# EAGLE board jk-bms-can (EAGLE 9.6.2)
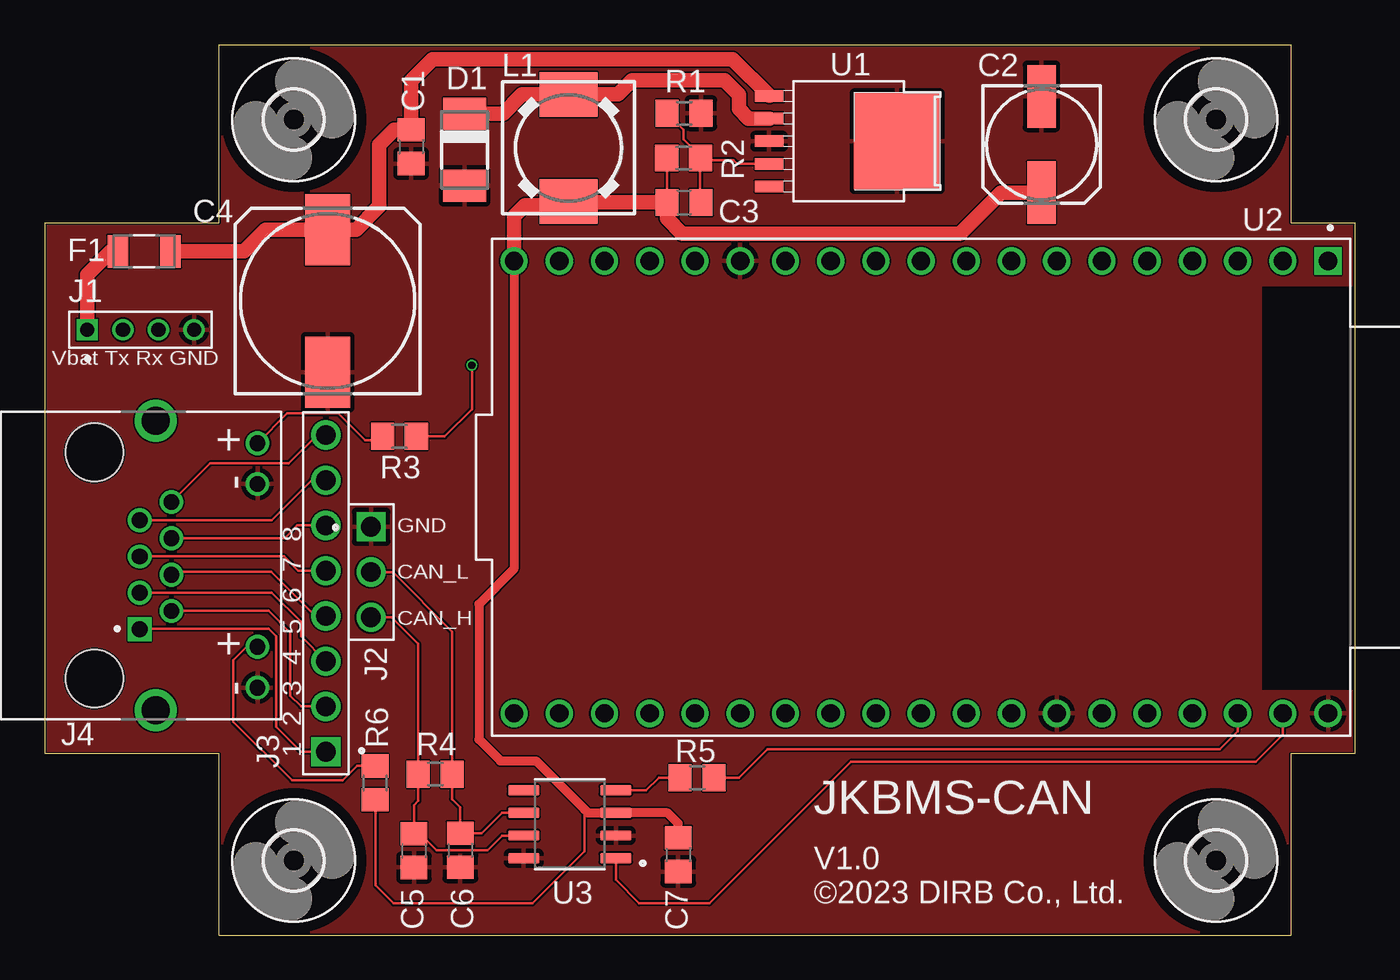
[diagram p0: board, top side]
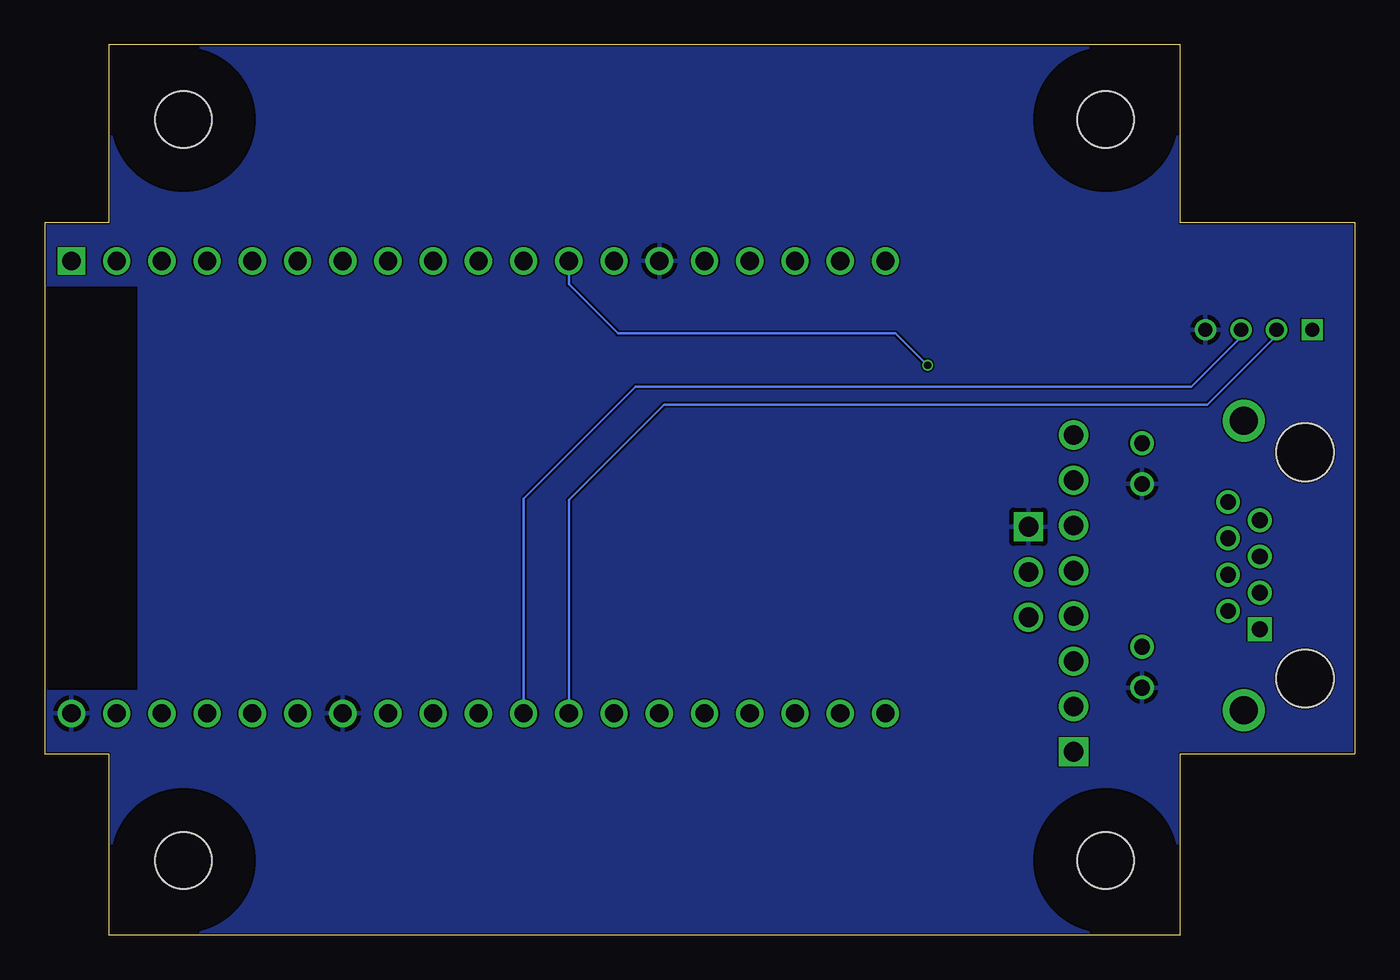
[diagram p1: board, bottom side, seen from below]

Size 73.6 x 50 mm. Coordinates in mm from the lower left corner, seen from the top.
Outline: 9.8,0 70,0 70,10.2 73.6,10.2 73.6,40 70,40 70,50 9.8,50 9.8,40 0,40 0,10.2 9.8,10.2 9.8,0
Copper layers (1*16): Top 0.035mm / dielectric 0.2mm / Bottom 0.035mm
Design rules "jlcpcb-2-layer": minimum track width 3.5mil, minimum drill 0.2mm, track to track 3.5mil, track to pad 5mil, pad to pad 5mil, via to via 5mil, smd to smd 0mil, copper to edge 0.1mm, drill to drill 5mil, minimum pad ring 4mil, minimum via ring 4mil, stop-mask expansion 3mil, vias tented up to drill 100mil, thermal gap 10mil
tRestrict: area 68.4,13.8 to 73.4,36.4
bRestrict: area 68.4,13.8 to 73.4,36.4

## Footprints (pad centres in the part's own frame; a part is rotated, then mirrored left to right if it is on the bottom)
C0805 = smd 1.3 x 1.5: 1 -0.95,0; 2 0.95,0
153CLV-0605 = smd 3.5 x 1.6: + 2.7,0; - -2.7,0
153CLV-1010 = smd 4 x 2.5: + 4,0; - -4,0
DO-214AC = smd 1.8 x 2.4: A 2.025,0; C -2.025,0
FUSC3216X75N = smd 1.16 x 1.82: 1 -1.475,0; 2 1.475,0
3,2 = hole 3.2: 0,0
62000411121 = drill 0.8 square: 1 -3,0 | drill 0.8: 2 -1,0; 3 1,0; 4 3,0
61300311121 = drill 1.1 square: 1 -2.54,0 | drill 1.1: 2 0,0; 3 2.54,0
61300811121 = drill 1.1 square: 1 -8.89,0 | drill 1.1: 2 -6.35,0; 3 -3.81,0; 4 -1.27,0; 5 1.27,0; 6 3.81,0; 7 6.35,0; 8 8.89,0
TE_2-406549-1 = drill 0.89 square: 1 0,0 | drill 0.89: 2 -1.02,1.78; 3 -2.04,0; 4 -3.06,1.78; 5 -4.08,0; 6 -5.1,1.78; 7 -6.12,0; 8 -7.14,1.78; 9 3.28,6.61; 10 0.99,6.61; 11 -8.15,6.61; 12 -10.44,6.61 | drill 1.57: S1 -11.71,0.89; S2 4.55,0.89 | hole 3.25: -9.93,-2.54; 2.77,-2.54
DR74 = smd 2.5 x 3.25: 1 -3,0; 2 3,0
R0805 = smd 1.3 x 1.5: 1 -0.95,0; 2 0.95,0
TO-252-5L = smd 0.65 x 1.6: 1 -2.535,-4.465; 2 -1.265,-4.465; 3 0.005,-4.47; 4 1.275,-4.47; 5 2.545,-4.47 | smd 5.42 x 4.84: 6/GND 0,2.715
MODULE_ESP32-DEVKITC-32U = drill 1.02 square: 1 -12.7,22.85 | drill 1.02: 2 -12.7,20.31; 3 -12.7,17.77; 4 -12.7,15.23; 5 -12.7,12.69; 6 -12.7,10.15; 7 -12.7,7.61; 8 -12.7,5.07; 9 -12.7,2.53; 10 -12.7,-0.01; 11 -12.7,-2.55; 12 -12.7,-5.09; 13 -12.7,-7.63; 14 -12.7,-10.17; 15 -12.7,-12.71; 16 -12.7,-15.25; 17 -12.7,-17.79; 18 -12.7,-20.33; 19 -12.7,-22.87; 20 12.7,-22.87; 21 12.7,-20.33; 22 12.7,-17.79; 23 12.7,-15.25; 24 12.7,-12.71; 25 12.7,-10.17; 26 12.7,-7.63; 27 12.7,-5.09; 28 12.7,-2.55; 29 12.7,-0.01; 30 12.7,2.53; 31 12.7,5.07; 32 12.7,7.61; 33 12.7,10.15; 34 12.7,12.69; 35 12.7,15.23; 36 12.7,17.77; 37 12.7,20.31; 38 12.7,22.85
SOIC127P600X175-8N = smd 1.75 x 0.59: 1 -2.585,1.905; 2 -2.585,0.635; 3 -2.585,-0.635; 4 -2.585,-1.905; 5 2.585,-1.905; 6 2.585,-0.635; 7 2.585,0.635; 8 2.585,1.905

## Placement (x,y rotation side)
C1  100n  [C0805]  20.59,44.28 270 top
C2  100uF/25V  [153CLV-0605]  56,44.4 270 top
C3  33n  [C0805]  35.92,41.15 0 top
C4  33uF/100V  [153CLV-1010]  15.9,35.62 90 top
C5  30p  [C0805]  20.75,4.76 270 top
C6  30p  [C0805]  23.35,4.78 270 top
C7  100n  [C0805]  35.59,4.53 270 top
D1  SS210  [DO-214AC]  23.59,44.1 270 top
F1  1206L035YR  [FUSC3216X75N]  5.6,38.4 0 top
H1  MOUNT-HOLE3.2  [3,2]  14,45.8 0 top
H2  MOUNT-HOLE3.2  [3,2]  65.8,45.8 0 top
H3  MOUNT-HOLE3.2  [3,2]  14,4.2 0 top
H4  MOUNT-HOLE3.2  [3,2]  65.8,4.2 0 top
J1  62000411121  [62000411121]  5.4,34 0 top
J2  61300311121  [61300311121]  18.34,20.4 270 top
J3  61300811121  [61300811121]  15.8,19.2 90 top
J4  2-406549-1  [TE_2-406549-1]  5.35,17.19 270 top
L1  470uH/0.5A  [DR74]  29.43,44.21 270 top
R1  10k  [R0805]  35.92,46.15 180 top
R2  30k  [R0805]  35.9,43.65 180 top
R3  10k  [R0805]  19.93,28.02 180 top
R4  120  [R0805]  21.94,9.05 180 top
R5  4K7  [R0805]  36.65,8.85 0 top
R6  10k  [R0805]  18.57,8.56 90 top
U1  XL7015  [TO-252-5L]  45.17,44.59 270 top
U2  ESP32-DEVKITC-32U  [MODULE_ESP32-DEVKITC-32U]  49.24,25.16 270 top
U3  TJA1050T/CM,118  [SOIC127P600X175-8N]  29.5,6.24 180 top

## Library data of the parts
C1-C7 = rcl; SPICEPREFIX: C
D1 = diode
F1 = 1206L035YR; AVAILABILITY: In Stock; CHECK_PRICES: https://www.snapeda.com/parts/1206L035YR/Littelfuse/view-part/?ref=eda; DESCRIPTION: PTC Resettable Fuse 0.35A(hold) 0.75A(trip) 6VDC 100A 0.6W 0.1s 0.3Ohm SMD Solder Pad 1206 T/R; MF: Littelfuse; MP: 1206L035YR; PACKAGE: None; PRICE: None; PURCHASE-URL: https://pricing.snapeda.com/search?q=1206L035YR&ref=eda; SNAPEDA_LINK: https://www.snapeda.com/parts/1206L035YR/Littelfuse/view-part/?ref=snap
H1-H4 = holes
J1 = Headers; CREATED_BY: PCBLayout.com; MANUFACTURER: Würth Elektronik; MPN: 62000411121
J2 = Headers; CREATED_BY: PCBLayout.com; DIGI_KEY_PART_NUMBER: 732-5316-ND; MANUFACTURER: Wurth Electronics Inc.; MPN: 61300311121
J3 = Headers; CREATED_BY: PCBLayout.com; DIGI_KEY_PART_NUMBER: 732-5321-ND; MANUFACTURER: Wurth Electronics Inc.; MPN: 61300811121
J4 = 2-406549-1; AVAILABILITY: In Stock; CENTERLINE_PITCH: 1.02 mm[.04 in]; CHECK_PRICES: https://www.snapeda.com/parts/2-406549-1/TE+Connectivity+AMP+Connectors/view-part/?ref=eda; COMMENT: 2-406549-1; DESCRIPTION: Jack Modular Connector 8p8c (RJ45, Ethernet) 90° Angle (Right) Shielded, EMI Finger Cat5; EU_ROHS_COMPLIANCE: Compliant; MF: TE Connectivity; MP: 2-406549-1; NUMBER_OF_POSITIONS: 8; PACKAGE: None; PRICE: None; PURCHASE-URL: https://pricing.snapeda.com/search?q=2-406549-1&ref=eda; SNAPEDA_LINK: https://www.snapeda.com/parts/2-406549-1/TE+Connectivity+AMP+Connectors/view-part/?ref=snap
L1 = inductors; SPICEPREFIX: L
R1-R6 = rcl; SPICEPREFIX: R
U1 = XL7015; AVAILABILITY: Not in stock; CHECK_PRICES: https://www.snapeda.com/parts/XL7015/XLSEMI/view-part/?ref=eda; DESCRIPTION: 0.8A 150KHz 80V Buck DC to DC; MF: XLSEMI; MP: XL7015; PACKAGE: Package; PRICE: None; SNAPEDA_LINK: https://www.snapeda.com/parts/XL7015/XLSEMI/view-part/?ref=snap
U2 = ESP32-DEVKITC-32U; AVAILABILITY: In Stock; CHECK_PRICES: https://www.snapeda.com/parts/ESP32-DEVKITC-32U/Espressif+Systems/view-part/?ref=eda; DESCRIPTION: ESP32-WROOM-32UE series Transceiver; 802.11 b/g/n (Wi-Fi, WiFi, WLAN), Bluetooth® Smart Ready 4.x Dual Mode Evaluation Board; MF: Espressif Systems; MP: ESP32-DEVKITC-32U; PACKAGE: CUSTOM-38 ESPRESSIF; PRICE: None; PURCHASE-URL: https://pricing.snapeda.com/search?q=ESP32-DEVKITC-32U&ref=eda; SNAPEDA_LINK: https://www.snapeda.com/parts/ESP32-DEVKITC-32U/Espressif+Systems/view-part/?ref=snap
U3 = TJA1050T_CM_118; AVAILABILITY: In Stock; CHECK_PRICES: https://www.snapeda.com/parts/TJA1050T/CM,118/NXP+USA+Inc./view-part/?ref=eda; DESCRIPTION: 1/1 Transceiver Half CANbus 8-SO; MF: NXP USA; MP: TJA1050T/CM,118; PACKAGE: SO-8 NXP Semiconductors; PRICE: None; PURCHASE-URL: https://pricing.snapeda.com/search?q=TJA1050T/CM,118&ref=eda; SNAPEDA_LINK: https://www.snapeda.com/parts/TJA1050T/CM,118/NXP+USA+Inc./view-part/?ref=snap

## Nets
3V3: U2.1
CAN_RXD: R5.1 U3.4
CAN_TXD: U2.37 U3.1
GND: C1.2 C2.- C4.- C5.2 C6.2 C7.2 D1.A J1.4 J2.1 J4.9 J4.11 R1.1 U1.3 U1.6/GND U2.14 U2.32 U2.38 U3.2 U3.8
JKBMS_RX: J1.3 U2.28
JKBMS_TX: J1.2 U2.27
LED_GRN: J4.10 R6.2
LED_YLW: J4.12 R3.2
N$1: F1.1 J1.1
N$3: C6.1 J2.2 R4.1 U3.6
N$4: C5.1 J2.3 R4.2 U3.7
N$5: C1.1 C4.+ F1.2 U1.1
N$7: C3.2 R1.2 R2.1 U1.4
N$8: R5.2 U2.36
N$9: J3.8 J4.8
N$10: J3.7 J4.7
N$11: J3.6 J4.6
N$12: D1.C L1.1 U1.2
N$13: J3.5 J4.5
N$14: J3.4 J4.4
N$15: J3.3 J4.3
N$16: J3.2 J4.2
N$17: J3.1 J4.1
N$22: R3.1 U2.12
VCC: C2.+ C3.1 C7.1 L1.2 R2.2 R6.1 U2.19 U3.3

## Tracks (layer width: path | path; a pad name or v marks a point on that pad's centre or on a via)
CAN_RXD
  Top 0.15: U3.4 33.8,8.14 34.5,8.85 R5.1
CAN_TXD
  Top 0.15: U2.37 69.55,11.26 68.03,9.74 45.29,9.74 37.35,1.8 33.4,1.8 32.09,3.12 U3.1
GND
  pour Top: 9.8,50 70,50 70,40 73.6,40 73.6,10.2 70.2,10.2 70.2,10 70,10 70,0 9.8,0 9.8,10.2 0,10.2 0,40 9.8,40
  pour Bottom: 70,50 70,40 73.6,40 73.6,10.2 70,10.2 70,0 9.8,0 9.8,10 9.8,10.2 0,10.2 0,40 9.8,40 9.8,50 10,50
JKBMS_RX
  Bottom 0.15: U2.28 46.69,24.51 40.4,30.8 9.18,30.8 6.4,33.58 J1.3
JKBMS_TX
  Bottom 0.15: U2.27 44.15,24.45 38.8,29.8 8.28,29.8 4.4,33.68 J1.2
LED_GRN
  Top 0.15: J4.10 11.36,16.2 10.6,15.44 10.6,12 13.91,8.69 16.75,8.69 17.57,9.51 R6.2
LED_YLW
  Top 0.15: J4.12 13.63,29.3 16.5,29.3 18,27.8 18.76,27.8 R3.2
N$1
  Top 0.813: J1.1 2.4,37.08 3.73,38.4 F1.1
N$3
  Top 0.15: U3.6 25.7,6.88 24.55,5.73 C6.1 23.35,7.19 22.89,7.65 R4.1 22.89,17.06 19.57,20.37 18.37,20.37 J2.2
N$4
  Top 0.15: U3.7 25.71,5.61 24.88,4.78 22.02,4.78 21.08,5.71 C5.1 20.75,7.31 20.99,7.55 R4.2 20.99,16.36 19.49,17.86 J2.3
N$5
  Top 0.813: F1.2 11.2,38.4 12.42,39.62 C4.+ 17.5,39.62 18.8,40.92 18.8,44.4 19.63,45.23 C1.1 20.59,47.99 21.8,49.2 38.63,49.2 U1.1
N$7
  Top 0.15: R1.2 35.9,45.22 35.9,44.7 36.85,43.75 R2.1 36.8,43.6 | 36.8,43.6 36.65,43.6 36.73,43.52 38.7,43.52 38.9,43.31 U1.4 | 36.8,43.6 36.8,41.16 C3.2
N$8
  Top 0.15: R5.2 39,8.85 40.6,10.45 66,10.45 67.01,11.46 U2.36
N$9
  Top 0.15: J4.8 9.3,26.5 13.71,26.5 15.3,28.09 J3.8
N$10
  Top 0.15: J3.7 15,25.55 12.76,23.31 J4.7
N$11
  Top 0.15: J3.6 14.2,23.01 13.48,22.29 J4.6
N$12
  Top 0.813: D1.C 25.75,46.12 26.83,47.21 L1.1 32.21,47.21 33,48 38.2,48 39,47.2 39,46.4 39.55,45.85 U1.2
N$13
  Top 0.15: J4.5 13.45,21.27 14.25,20.47 J3.5
N$14
  Top 0.15: J3.4 15.2,17.93 12.73,20.4 7.28,20.4 J4.4
N$15
  Top 0.15: J3.3 14.4,16.79 14.4,17.6 12.77,19.23 J4.3
N$16
  Top 0.15: J3.2 14.4,12.85 13.8,13.45 13.8,17 12.59,18.21 J4.2
N$17
  Top 0.15: J4.1 12.6,17.2 13,16.8 13,11.71 14.4,10.31 J3.1
N$22  (via drill 0.4)
  Top 0.15: R3.1 22.48,28.02 24,29.54 v24,32
  Bottom 0.15: v24,32 25.8,33.8 41.4,33.8 44.15,36.55 U2.12
VCC
  Top 0.15: R2.2 34.95,41.19 | 34.95,41.19 34.95,40.99 | 34.95,41.19 C3.1 | R6.1 18.6,7.58 18.6,2.8 19.6,1.8 27.4,1.8 30.32,4.72 30.32,7.08
  Top 0.508: C7.1 35.59,6.28 34.99,6.88 U3.3 30.52,6.88 30.32,7.08 27.6,9.8 25.6,9.8 24.4,11 24.4,18.6 26.37,20.57 U2.19
  Top 0.813: C2.+ 53.7,41.7 51.4,39.4 35.8,39.4 34.95,40.25 34.95,40.99 | C3.1 29.49,41.15 L1.2 29.22,41 27,41 26.37,40.37 U2.19

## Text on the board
tNames: Vbat Tx Rx GND | GND | CAN_L | CAN_H | 1 2 3 4 5 6 7 8 | JKBMS-CAN | V1.0 / ©2023 DIRB Co., Ltd.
